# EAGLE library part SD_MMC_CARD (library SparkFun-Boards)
SD MMC Card Footprint Mechanical footprint with connectors of an SD/MMC card- NOT a socket! SparkFun Products: Electric Imp microSD Card with SD adapter
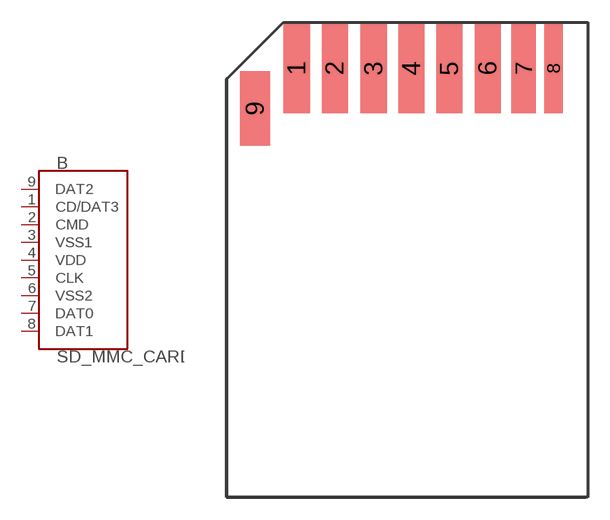
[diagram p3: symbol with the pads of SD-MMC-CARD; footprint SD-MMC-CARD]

Designator prefix B

## SD_MMC_CARDSD_PCB  [SD-MMC-CARD]
1  CD/DAT3
2  CMD
3  VSS1
4  VDD
5  CLK
6  VSS2
7  DAT0
8  DAT1
9  DAT2

## Footprint SD-MMC-CARD (pad centres in mm)
SD MMC Card Footprint Basic reference with pads for SMD mounting of SD card. Specifications: Pin count:9 Area:0.95x1.25 inch Example device(s): SD Card
smd 1.75 x 6: 1 -8.015,14.713; 2 -5.465,14.703; 3 -2.87,14.703; 4 -0.34,14.703; 5 2.195,14.703; 6 4.76,14.703
smd 1.65 x 6: 7 7.16,14.703
smd 1.25 x 6: 8 9.16,14.703
smd 2 x 5: 9 -10.8,12.03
